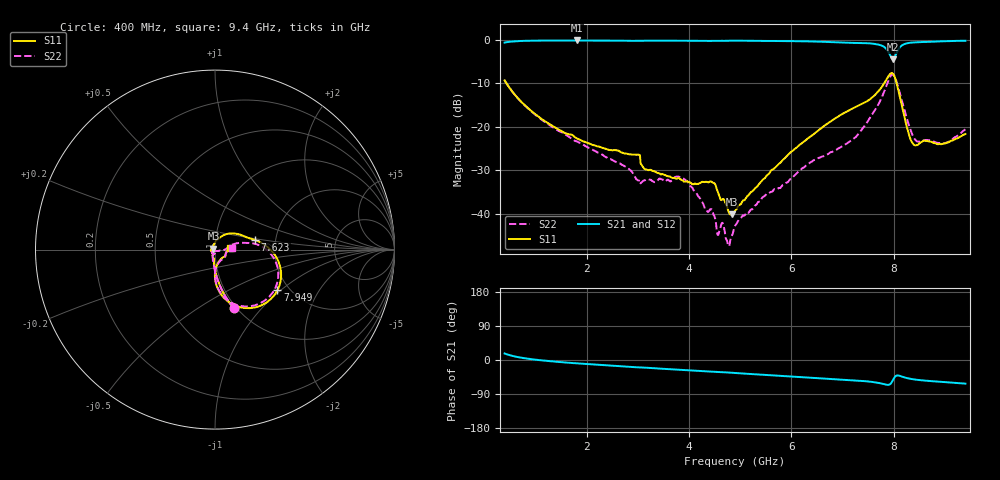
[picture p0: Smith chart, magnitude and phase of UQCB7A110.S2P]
!  Part Number  UQCB7A110	Mounting Orientation: Vertical
!  Description: RF capacitors
!  Application: Coupling, Bypass, Tuning, DC Block
!  Filters, Matching
# GHZ S DB R 50
! Freq  |S11|  S11 Ph  |S21|  S21 Ph  |S12|  S12 Ph  |S22|  S22 Ph
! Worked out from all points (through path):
!   801 points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, 400 MHz to 9.4 GHz, reference 50 ohm
!   highest |S21| = -0.09 dB at 1.806 GHz (marker M1); lowest = -4.4 dB at 7.983 GHz (marker M2)
!   group delay of S21, straight-line fit = 21.2 ps
!   lowest |S11| = -40.2 dB at 4.844 GHz (marker M3), VSWR 1.02, Z = 49.2 + j0.478 ohm
!   |S11| at or under -10 dB: 437.9 MHz to 7.812 GHz (7.375 GHz wide, 179 % of centre); 8.057 GHz to end of sweep
!   |S22| runs from -47.5 to -7.9 dB; largest |S21 - S12| = 0.0046
!   S11 on the Smith chart (normalised r, x): 400 MHz: 0.97, -0.72; 7.623 GHz: 1.56, +0.18; 7.949 GHz: 1.74, -0.95; 9.4 GHz: 1.18, +0.02
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0.4  -9.29 -72.3  -0.58 17.2  -0.56 17.2  -9.28 -72.2
0.996  -17.05 -87.3  -0.13 0.9  -0.12 0.9  -17.17 -88.0
1.806  -22.63 -94.5  -0.09 -8.8  -0.08 -8.9  -23.34 -98.3
1.908  -23.21 -94.5  -0.10 -9.8  -0.08 -9.9  -23.98 -100.2
3.033  -26.45 -102.5  -0.20 -19.3  -0.18 -19.4  -32.34 -113.3
3.404  -30.62 -113.3  -0.12 -22.5  -0.10 -22.6  -32.16 -99.9
3.91  -32.64 -128.6  -0.15 -26.7  -0.14 -26.8  -32.08 -131.0
4.461  -32.83 -176.4  -0.20 -30.9  -0.19 -31.0  -39.50 -139.9
4.563  -34.93 160.1  -0.19 -31.4  -0.18 -31.5  -44.91 -128.8
4.754  -38.77 142.5  -0.16 -32.9  -0.15 -33.0  -46.78 -102.2
4.844  -40.20 150.2  -0.14 -33.7  -0.13 -33.9  -44.97 -67.4
4.9  -39.36 151.9  -0.13 -34.3  -0.13 -34.4  -42.82 -57.8
6.408  -21.94 64.5  -0.32 -47.0  -0.33 -47.1  -27.95 -7.2
7.218  -15.65 29.9  -0.65 -53.6  -0.66 -53.8  -22.73 9.5
7.623  -12.79 13.5  -0.87 -58.7  -0.88 -58.9  -16.35 14.5
7.904  -8.20 -18.9  -2.89 -65.4  -2.90 -65.6  -9.12 -12.5
7.949  -7.63 -33.1  -3.96 -61.3  -3.97 -61.5  -8.14 -27.3
7.983  -7.72 -46.1  -4.40 -53.7  -4.42 -53.9  -7.95 -40.8
8.129  -13.53 -86.6  -1.54 -42.4  -1.56 -42.6  -12.65 -83.8
8.399  -24.19 -56.9  -0.54 -51.3  -0.55 -51.5  -22.61 -72.1
9.006  -23.82 -10.1  -0.27 -58.5  -0.28 -58.7  -23.72 -15.7
9.4  -21.65 5.8  -0.16 -62.4  -0.18 -62.5  -20.58 5.3
